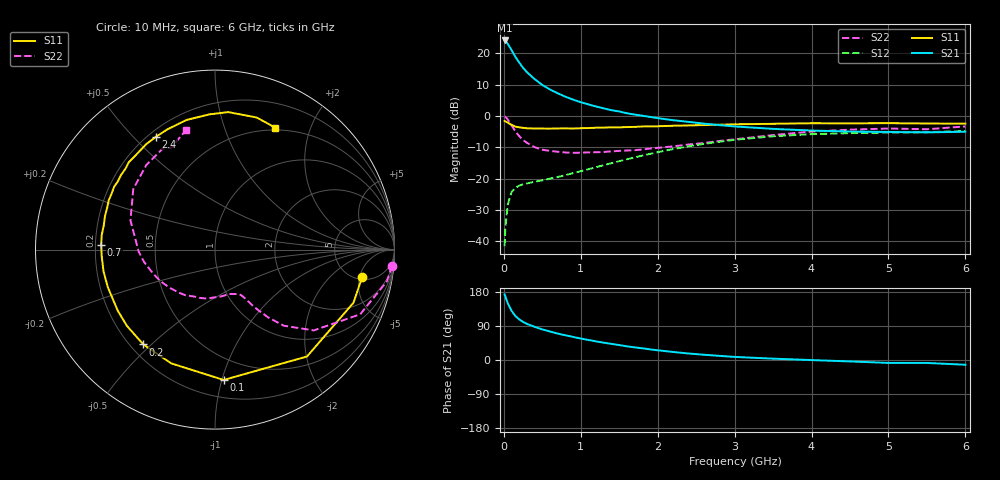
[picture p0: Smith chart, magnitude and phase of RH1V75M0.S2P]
! SIEMENS Small Signal Semiconductors
! BFR106
! Si NPN RF Bipolar Junction Transistor in SOT23
! VCE = 1.75 V  IC = 5 mA
! Common Emitter S-Parameters:  August  1996
# GHz  S  MA  R  50
!  f  S11  S21  S12  S22
! GHz  MAG  ANG  MAG  ANG  MAG  ANG  MAG  ANG
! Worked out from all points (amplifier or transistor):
!   36 points, 10 MHz to 6 GHz, reference 50 ohm
!   highest |S21| = 24.1 dB at 10 MHz (marker M1)
!   |S21| within 3 dB of that: start of sweep to 98.36 MHz
!   unconditionally stable (mu >= 1): 606.2 MHz to 2.269 GHz; 4.125 GHz to end of sweep
!   at 250 MHz: K = 0.51, MSG = 18.6 dB, |S12| = -21.8 dB
!   at 1.4 GHz: K = 1.17, MAG = 6.0 dB, |S12| = -15.0 dB
!   at 6 GHz: K = 1.03, MAG = -1.1 dB, |S12| = -4.8 dB
!   S11 on the Smith chart (normalised r, x): 10 MHz: 5.38, -5.48; 100 MHz: 0.33, -1.01; 200 MHz: 0.25, -0.47; 700 MHz: 0.22, +0.02; 2.4 GHz: 0.23, +0.58; 6 GHz: 0.47, +1.50
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0.01  0.8341 -10.7  16.11 172.9  0.0084 86.8  0.9896 -5.2
0.02  0.8263 -21.0  15.88 167.5  0.0165 80.1  0.9742 -10.4
0.05  0.7857 -49.3  14.29 150.1  0.0384 64.8  0.8858 -24.0
0.1  0.7279 -86.2  11.32 130.1  0.0613 50.1  0.7109 -39.3
0.15  0.6792 -111.0  8.82 116.0  0.0717 41.2  0.5714 -47.9
0.2  0.6622 -127.1  7.145 107.3  0.0778 37.5  0.48 -51.9
0.25  0.6492 -139.1  5.897 100.4  0.0816 35.4  0.4145 -54.5
0.3  0.6398 -147.9  5.033 95.4  0.0842 35.0  0.3751 -56.1
0.4  0.6329 -160.7  3.886 87.5  0.0895 35.7  0.3194 -58.3
0.5  0.6329 -168.9  3.14 80.8  0.0942 37.8  0.2908 -60.3
0.6  0.6322 -176.4  2.654 75.1  0.1006 40.5  0.2784 -62.9
0.7  0.6352 177.5  2.315 69.8  0.1067 43.2  0.2697 -66.6
0.9  0.6341 167.7  1.832 60.9  0.1229 48.1  0.2588 -73.8
1.1  0.6445 158.8  1.537 52.8  0.1421 52.0  0.2634 -83.0
1.3  0.6555 151.2  1.327 45.7  0.1652 54.3  0.2675 -92.4
1.6  0.6684 141.5  1.109 36.1  0.2047 55.7  0.2825 -107.9
2.2  0.7014 123.1  0.86 21.2  0.2976 51.4  0.3288 -139.2
2.4  0.7097 117.5  0.809 17.1  0.3296 48.8  0.3526 -150.3
3.5  0.7538 92.5  0.625 3.5  0.4766 29.0  0.4984 160.9
4.5  0.7666 78.1  0.567 -3.8  0.5346 11.3  0.6073 129.0
5.5  0.7617 67.5  0.55 -7.8  0.5545 0.9  0.6171 113.5
6  0.7576 63.7  0.563 -12.5  0.5776 -6.4  0.6836 103.8
